| TEXAS INSTRUMENTS INCORPORATED
| Standard Linear and Logic Group
| IBIS Model of SN74CBTLV16211
| LOW-VOLTAGE 24-BIT FET BUS SWITCH
| This file contains package information for the following:
|  TVSOP 56-pin (DGV) package as [Component] CBTLV16211_DGV
|  TSSOP 56-pin (DGG) package as [Component] CBTLV16211_DGG
|  SSOP 56-pin (DL) package as [Component] CBTLV16211_DL
| This device can be powered at the following Vccs:
|  3.3 volt Vcc
|  2.5 volt Vcc
| This file provides unique models under the [Model Selector] for each Vcc.
| For operation at a specific Vcc, select the appropriate model after each
| [Model Selector] keyword.
[IBIS Ver]   3.2
[Comment char]  |_char
[File Name]   sn74cbtlv16211.ibs
[File Rev]   1.1 | b_die
[Date]   December 16, 2002
[Source]   Data created from TI-SPICE simulations at TI-SLL.
[Notes]   The following is an IBIS list for the CBTLV16211.
   Please contact sllibis@ti.com with questions and
   comments concerning SLL IBIS models.
   -Power clamp data deleted as there is no power-clamp diode.
   -Non-monotonic data due to FET characteristics.
[Disclaimer] Property of Texas Instruments Incorporated.  Unauthorized
   reproduction and/or distribution is strictly prohibited.
   This product is protected under copyright law.
   Created  2002, (C) Copyright  2002, Texas Instruments
   Incorporated, All Rights Reserved
   UNLESS THERE IS A SIGNED, WRITTEN AGREEMENT TO THE
   CONTRARY, TEXAS INSTRUMENTS (TI) IS PROVIDING THE IBIS
   MODELS  AND WITHOUT ANY WARRANTY, EXPRESSED OR
   IMPLIED.  TI assumes no liability for:
   1) the accuracy of the IBIS models provided to your
   company;
   2) the proper functioning of these IBIS Models in your
   design or for any resulting applications; or
   3) infringement of patents, copyrights or intellectual
   property rights resulting from your use of these IBIS
   models.
   TI provides IBIS Models as a service to our customers.
   You and your company shall not distribute, sell or give
   these models to anyone else without prior written
   permission from TI.
   TI reserves the right to make changes to our products or
   to discontinue any semiconductor product or service
   without notice, and advises our customers to obtain the
   latest version of relevant information to verify, before
   placing orders, that the information being relied on is
   current.
   Please be aware that your receipt and use of the IBIS
   information provided shall serve as acceptance of these
   terms and conditions.  If you do not accept these terms,
   you should return or destroy the IBIS models and any
   other accompanying information immediately.
| Component CBTLV16211_DGV 56-pin TVSOP
[Component]   CBTLV16211_DGV
[Manufacturer]   Texas Instruments, Inc.
[Package]
|   typ   min   max
R_pkg   6.300e-02   5.000e-02   8.600e-02
L_pkg   2.945e-09   2.392e-09   3.938e-09
C_pkg   3.910e-13   2.710e-13   5.880e-13
[Pin]   signal_name   model_name   R_pin   L_pin   C_pin
1   NC   NC   6.800e-02   3.933e-09   5.880e-13
2   1A1   CBTLV16211_IO   6.800e-02   3.569e-09   5.860e-13
3   1A2   CBTLV16211_IO   7.600e-02   3.464e-09   5.150e-13
4   1A3   CBTLV16211_IO   8.600e-02   3.451e-09   4.580e-13
5   1A4   CBTLV16211_IO   8.200e-02   3.278e-09   4.260e-13
6   1A5   CBTLV16211_IO   7.700e-02   3.143e-09   3.870e-13
7   1A6   CBTLV16211_IO   6.900e-02   2.971e-09   4.010e-13
8   GND   GND   5.000e-02   2.787e-09   3.790e-13
9   1A7   CBTLV16211_IO   5.100e-02   2.686e-09   3.200e-13
10   1A8   CBTLV16211_IO   5.200e-02   2.607e-09   3.160e-13
11   1A9   CBTLV16211_IO   5.300e-02   2.497e-09   2.970e-13
12   1A10   CBTLV16211_IO   5.400e-02   2.438e-09   2.920e-13
13   1A11   CBTLV16211_IO   5.500e-02   2.412e-09   2.860e-13
14   1A12   CBTLV16211_IO   5.500e-02   2.400e-09   2.730e-13
15   2A1   CBTLV16211_IO   5.500e-02   2.402e-09   2.730e-13
16   2A2   CBTLV16211_IO   5.400e-02   2.398e-09   2.840e-13
17   VCC   POWER   5.400e-02   2.407e-09   2.890e-13
18   2A3   CBTLV16211_IO   5.300e-02   2.448e-09   2.930e-13
19   GND   GND   5.200e-02   2.548e-09   3.110e-13
20   2A4   CBTLV16211_IO   5.100e-02   2.623e-09   3.160e-13
21   2A5   CBTLV16211_IO   5.000e-02   2.725e-09   3.700e-13
22   2A6   CBTLV16211_IO   6.500e-02   2.903e-09   3.940e-13
23   2A7   CBTLV16211_IO   7.300e-02   3.086e-09   3.870e-13
24   2A8   CBTLV16211_IO   8.200e-02   3.272e-09   4.280e-13
25   2A9   CBTLV16211_IO   8.200e-02   3.394e-09   4.570e-13
26   2A10   CBTLV16211_IO   7.100e-02   3.374e-09   5.080e-13
27   2A11   CBTLV16211_IO   6.900e-02   3.572e-09   5.810e-13
28   2A12   CBTLV16211_IO   6.900e-02   3.937e-09   5.740e-13
29   2B12   CBTLV16211_IO   6.900e-02   3.923e-09   5.690e-13
30   2B11   CBTLV16211_IO   6.800e-02   3.546e-09   5.740e-13
31   2B10   CBTLV16211_IO   7.400e-02   3.422e-09   5.180e-13
32   2B9   CBTLV16211_IO   8.100e-02   3.395e-09   4.680e-13
33   2B8   CBTLV16211_IO   8.000e-02   3.255e-09   4.310e-13
34   2B7   CBTLV16211_IO   7.100e-02   3.063e-09   3.860e-13
35   2B6   CBTLV16211_IO   6.100e-02   2.878e-09   3.900e-13
36   2B5   CBTLV16211_IO   5.000e-02   2.709e-09   3.640e-13
37   2B4   CBTLV16211_IO   5.100e-02   2.607e-09   3.110e-13
38   GND   GND   5.100e-02   2.532e-09   3.060e-13
39   2B3   CBTLV16211_IO   5.300e-02   2.440e-09   2.890e-13
40   2B2   CBTLV16211_IO   5.300e-02   2.399e-09   2.860e-13
41   2B1   CBTLV16211_IO   5.400e-02   2.392e-09   2.820e-13
42   1B12   CBTLV16211_IO   5.500e-02   2.399e-09   2.710e-13
43   1B11   CBTLV16211_IO   5.500e-02   2.395e-09   2.710e-13
44   1B10   CBTLV16211_IO   5.500e-02   2.403e-09   2.830e-13
45   1B9   CBTLV16211_IO   5.400e-02   2.421e-09   2.880e-13
46   1B8   CBTLV16211_IO   5.300e-02   2.472e-09   2.920e-13
47   1B7   CBTLV16211_IO   5.100e-02   2.569e-09   3.090e-13
48   1B6   CBTLV16211_IO   5.100e-02   2.636e-09   3.130e-13
49   GND   GND   5.000e-02   2.739e-09   3.660e-13
50   1B5   CBTLV16211_IO   6.500e-02   2.922e-09   3.900e-13
51   1B4   CBTLV16211_IO   7.200e-02   3.076e-09   3.840e-13
52   1B3   CBTLV16211_IO   8.100e-02   3.249e-09   4.300e-13
53   1B2   CBTLV16211_IO   8.300e-02   3.400e-09   4.550e-13
54   1B1   CBTLV16211_IO   7.300e-02   3.421e-09   5.060e-13
55   2NOE   CBTLV16211_NOE   6.900e-02   3.579e-09   5.780e-13
56   1NOE   CBTLV16211_NOE   6.900e-02   3.938e-09   5.810e-13
| Component CBTLV16211_DGG 56-pin TSSOP
[Component]   CBTLV16211_DGG
[Manufacturer]   Texas Instruments, Inc.
[Package]
|   typ   min   max
R_pkg   4.500e-02   3.500e-02   6.200e-02
L_pkg   3.324e-09   2.403e-09   5.094e-09
C_pkg   5.640e-13   3.410e-13   9.140e-13
[Pin]   signal_name   model_name   R_pin   L_pin   C_pin
1   NC   NC   6.200e-02   5.094e-09   8.560e-13
2   1A1   CBTLV16211_IO   6.100e-02   4.621e-09   9.020e-13
3   1A2   CBTLV16211_IO   6.000e-02   4.316e-09   8.020e-13
4   1A3   CBTLV16211_IO   5.900e-02   3.968e-09   6.980e-13
5   1A4   CBTLV16211_IO   5.700e-02   3.716e-09   6.490e-13
6   1A5   CBTLV16211_IO   4.200e-02   3.517e-09   6.520e-13
7   1A6   CBTLV16211_IO   4.100e-02   3.160e-09   5.700e-13
8   GND   GND   3.900e-02   2.981e-09   4.820e-13
9   1A7   CBTLV16211_IO   3.900e-02   2.809e-09   4.470e-13
10   1A8   CBTLV16211_IO   3.800e-02   2.715e-09   4.090e-13
11   1A9   CBTLV16211_IO   4.100e-02   2.675e-09   3.910e-13
12   1A10   CBTLV16211_IO   3.900e-02   2.536e-09   3.660e-13
13   1A11   CBTLV16211_IO   3.900e-02   2.457e-09   3.480e-13
14   1A12   CBTLV16211_IO   3.800e-02   2.411e-09   3.530e-13
15   2A1   CBTLV16211_IO   3.900e-02   2.456e-09   3.550e-13
16   2A2   CBTLV16211_IO   3.900e-02   2.471e-09   3.490e-13
17   VCC   POWER   4.000e-02   2.580e-09   3.700e-13
18   2A3   CBTLV16211_IO   3.800e-02   2.651e-09   3.890e-13
19   GND   GND   3.800e-02   2.739e-09   4.110e-13
20   2A4   CBTLV16211_IO   3.900e-02   2.838e-09   4.490e-13
21   2A5   CBTLV16211_IO   3.800e-02   2.988e-09   4.840e-13
22   2A6   CBTLV16211_IO   3.800e-02   3.105e-09   5.640e-13
23   2A7   CBTLV16211_IO   4.000e-02   3.427e-09   6.380e-13
24   2A8   CBTLV16211_IO   5.600e-02   3.654e-09   6.410e-13
25   2A9   CBTLV16211_IO   5.700e-02   3.932e-09   7.000e-13
26   2A10   CBTLV16211_IO   5.800e-02   4.257e-09   8.060e-13
27   2A11   CBTLV16211_IO   5.700e-02   4.580e-09   9.140e-13
28   2A12   CBTLV16211_IO   5.900e-02   5.038e-09   8.610e-13
29   2B12   CBTLV16211_IO   6.000e-02   5.058e-09   8.580e-13
30   2B11   CBTLV16211_IO   5.600e-02   4.543e-09   9.040e-13
31   2B10   CBTLV16211_IO   5.700e-02   4.240e-09   8.030e-13
32   2B9   CBTLV16211_IO   5.700e-02   3.929e-09   7.000e-13
33   2B8   CBTLV16211_IO   5.600e-02   3.616e-09   6.370e-13
34   2B7   CBTLV16211_IO   3.700e-02   3.368e-09   6.400e-13
35   2B6   CBTLV16211_IO   3.600e-02   3.024e-09   5.630e-13
36   2B5   CBTLV16211_IO   3.500e-02   2.876e-09   4.740e-13
37   2B4   CBTLV16211_IO   3.500e-02   2.745e-09   4.440e-13
38   GND   GND   3.700e-02   2.683e-09   4.050e-13
39   2B3   CBTLV16211_IO   3.800e-02   2.603e-09   3.820e-13
40   2B2   CBTLV16211_IO   3.800e-02   2.510e-09   3.620e-13
41   2B1   CBTLV16211_IO   3.600e-02   2.412e-09   3.410e-13
42   1B12   CBTLV16211_IO   3.800e-02   2.416e-09   3.490e-13
43   1B11   CBTLV16211_IO   3.700e-02   2.403e-09   3.490e-13
44   1B10   CBTLV16211_IO   3.700e-02   2.429e-09   3.410e-13
45   1B9   CBTLV16211_IO   3.600e-02   2.482e-09   3.580e-13
46   1B8   CBTLV16211_IO   3.700e-02   2.615e-09   3.810e-13
47   1B7   CBTLV16211_IO   3.500e-02   2.669e-09   4.020e-13
48   1B6   CBTLV16211_IO   3.600e-02   2.763e-09   4.420e-13
49   GND   GND   3.600e-02   2.942e-09   4.780e-13
50   1B5   CBTLV16211_IO   3.500e-02   3.053e-09   5.640e-13
51   1B4   CBTLV16211_IO   3.600e-02   3.409e-09   6.410e-13
52   1B3   CBTLV16211_IO   5.800e-02   3.698e-09   6.410e-13
53   1B2   CBTLV16211_IO   5.900e-02   3.975e-09   6.970e-13
54   1B1   CBTLV16211_IO   6.100e-02   4.327e-09   8.020e-13
55   2NOE   CBTLV16211_NOE   6.100e-02   4.624e-09   9.050e-13
56   1NOE   CBTLV16211_NOE   6.000e-02   5.063e-09   8.580e-13
| Component CBTLV16211_DL 56-pin SSOP
[Component]   CBTLV16211_DL
[Manufacturer]   Texas Instruments, Inc.
[Package]
|   typ   min   max
R_pkg   5.500e-02   4.800e-02   6.700e-02
L_pkg   6.539e-09   4.802e-09   9.746e-09
C_pkg   1.880e-13   7.600e-14   5.170e-13
[Pin]   signal_name   model_name   R_pin   L_pin   C_pin
1   NC   NC   6.400e-02   9.646e-09   5.130e-13
2   1A1   CBTLV16211_IO   5.900e-02   8.723e-09   2.700e-13
3   1A2   CBTLV16211_IO   5.900e-02   8.139e-09   2.230e-13
4   1A3   CBTLV16211_IO   5.600e-02   7.554e-09   2.010e-13
5   1A4   CBTLV16211_IO   5.400e-02   6.991e-09   1.950e-13
6   1A5   CBTLV16211_IO   5.300e-02   6.659e-09   2.020e-13
7   1A6   CBTLV16211_IO   5.500e-02   6.321e-09   2.070e-13
8   GND   GND   5.500e-02   5.942e-09   1.330e-13
9   1A7   CBTLV16211_IO   5.700e-02   5.767e-09   1.320e-13
10   1A8   CBTLV16211_IO   5.400e-02   5.459e-09   1.210e-13
11   1A9   CBTLV16211_IO   5.100e-02   5.224e-09   1.400e-13
12   1A10   CBTLV16211_IO   4.800e-02   5.088e-09   1.260e-13
13   1A11   CBTLV16211_IO   5.000e-02   5.021e-09   9.600e-14
14   1A12   CBTLV16211_IO   5.100e-02   4.802e-09   7.600e-14
15   2A1   CBTLV16211_IO   5.100e-02   4.803e-09   7.600e-14
16   2A2   CBTLV16211_IO   5.000e-02   5.021e-09   9.600e-14
17   VCC   POWER   4.800e-02   5.088e-09   1.260e-13
18   2A3   CBTLV16211_IO   5.100e-02   5.224e-09   1.400e-13
19   GND   GND   5.400e-02   5.459e-09   1.210e-13
20   2A4   CBTLV16211_IO   5.700e-02   5.768e-09   1.330e-13
21   2A5   CBTLV16211_IO   5.500e-02   5.942e-09   1.330e-13
22   2A6   CBTLV16211_IO   5.500e-02   6.320e-09   2.060e-13
23   2A7   CBTLV16211_IO   5.300e-02   6.659e-09   2.030e-13
24   2A8   CBTLV16211_IO   5.400e-02   6.991e-09   1.960e-13
25   2A9   CBTLV16211_IO   5.600e-02   7.554e-09   2.010e-13
26   2A10   CBTLV16211_IO   5.900e-02   8.139e-09   2.230e-13
27   2A11   CBTLV16211_IO   5.900e-02   8.727e-09   2.700e-13
28   2A12   CBTLV16211_IO   6.700e-02   9.746e-09   5.170e-13
29   2B12   CBTLV16211_IO   6.300e-02   9.630e-09   5.110e-13
30   2B11   CBTLV16211_IO   6.000e-02   8.751e-09   2.710e-13
31   2B10   CBTLV16211_IO   6.000e-02   8.184e-09   2.250e-13
32   2B9   CBTLV16211_IO   5.600e-02   7.543e-09   2.000e-13
33   2B8   CBTLV16211_IO   5.400e-02   7.005e-09   1.960e-13
34   2B7   CBTLV16211_IO   5.600e-02   6.714e-09   2.040e-13
35   2B6   CBTLV16211_IO   5.800e-02   6.384e-09   2.080e-13
36   2B5   CBTLV16211_IO   5.700e-02   5.976e-09   1.340e-13
37   2B4   CBTLV16211_IO   5.700e-02   5.743e-09   1.300e-13
38   GND   GND   5.400e-02   5.468e-09   1.190e-13
39   2B3   CBTLV16211_IO   5.500e-02   5.328e-09   1.420e-13
40   2B2   CBTLV16211_IO   5.200e-02   5.189e-09   1.290e-13
41   2B1   CBTLV16211_IO   5.200e-02   5.053e-09   9.600e-14
42   1B12   CBTLV16211_IO   5.100e-02   4.825e-09   7.600e-14
43   1B11   CBTLV16211_IO   5.400e-02   4.896e-09   7.800e-14
44   1B10   CBTLV16211_IO   5.200e-02   5.093e-09   9.700e-14
45   1B9   CBTLV16211_IO   5.100e-02   5.179e-09   1.280e-13
46   1B8   CBTLV16211_IO   5.400e-02   5.314e-09   1.420e-13
47   1B7   CBTLV16211_IO   5.500e-02   5.511e-09   1.210e-13
48   1B6   CBTLV16211_IO   5.700e-02   5.771e-09   1.310e-13
49   GND   GND   5.600e-02   5.957e-09   1.330e-13
50   1B5   CBTLV16211_IO   5.500e-02   6.320e-09   2.060e-13
51   1B4   CBTLV16211_IO   5.200e-02   6.621e-09   2.000e-13
52   1B3   CBTLV16211_IO   5.300e-02   6.973e-09   1.950e-13
53   1B2   CBTLV16211_IO   5.700e-02   7.571e-09   2.020e-13
54   1B1   CBTLV16211_IO   5.700e-02   8.097e-09   2.220e-13
55   2NOE   CBTLV16211_NOE   5.900e-02   8.723e-09   2.710e-13
56   1NOE   CBTLV16211_NOE   6.100e-02   9.560e-09   5.090e-13
[Series Switch Groups]
| Function Group States
On  1 /   | 1A1-1A12->1B1-1B12 1NOE LOW
On  2 /   | 2A1-2A12->2B1-2B12 2NOE LOW
On  1 2 /   | 1NOE, LOW, 2NOE, LOW
[Series Pin Mapping]   pin_2   model_name   function_table_group
2   54   CBTLV16211_IO_33_S   1
| 2   54   CBTLV16211_IO_25_S   1
3   53   CBTLV16211_IO_33_S   1
| 3   53   CBTLV16211_IO_25_S   1
4   52   CBTLV16211_IO_33_S   1
| 4   52   CBTLV16211_IO_25_S   1
5   51   CBTLV16211_IO_33_S   1
| 5   51   CBTLV16211_IO_25_S   1
6   50   CBTLV16211_IO_33_S   1
| 6   50   CBTLV16211_IO_25_S   1
7   48   CBTLV16211_IO_33_S   1
| 7   48   CBTLV16211_IO_25_S   1
9   47   CBTLV16211_IO_33_S   1
| 9   47   CBTLV16211_IO_25_S   1
10   46   CBTLV16211_IO_33_S   1
| 10   46   CBTLV16211_IO_25_S   1
11   45   CBTLV16211_IO_33_S   1
| 11   45   CBTLV16211_IO_25_S   1
12   44   CBTLV16211_IO_33_S   1
| 12   44   CBTLV16211_IO_25_S   1
13   43   CBTLV16211_IO_33_S   1
| 13   43   CBTLV16211_IO_25_S   1
14   42   CBTLV16211_IO_33_S   1
| 14   42   CBTLV16211_IO_25_S   1
15   41   CBTLV16211_IO_33_S   2
| 15   41   CBTLV16211_IO_25_S   2
16   40   CBTLV16211_IO_33_S   2
| 16   40   CBTLV16211_IO_25_S   2
18   39   CBTLV16211_IO_33_S   2
| 18   39   CBTLV16211_IO_25_S   2
20   37   CBTLV16211_IO_33_S   2
| 20   37   CBTLV16211_IO_25_S   2
21   36   CBTLV16211_IO_33_S   2
| 21   36   CBTLV16211_IO_25_S   2
22   35   CBTLV16211_IO_33_S   2
| 22   35   CBTLV16211_IO_25_S   2
23   34   CBTLV16211_IO_33_S   2
| 23   34   CBTLV16211_IO_25_S   2
24   33   CBTLV16211_IO_33_S   2
| 24   33   CBTLV16211_IO_25_S   2
25   32   CBTLV16211_IO_33_S   2
| 25   32   CBTLV16211_IO_25_S   2
26   31   CBTLV16211_IO_33_S   2
| 26   31   CBTLV16211_IO_25_S   2
27   30   CBTLV16211_IO_33_S   2
| 27   30   CBTLV16211_IO_25_S   2
28   29   CBTLV16211_IO_33_S   2
| 28   29   CBTLV16211_IO_25_S   2
| Model CBTLV16211_NOE
[Model Selector]   CBTLV16211_NOE
CBTLV16211_NOE_33   3.3 volt Vcc
CBTLV16211_NOE_25   2.5 volt Vcc
| Model CBTLV16211_IO
[Model Selector]   CBTLV16211_IO
CBTLV16211_IO_33   3.3 volt Vcc
CBTLV16211_IO_25   2.5 volt Vcc
| Model CBTLV16211_IO_S
[Model Selector]   CBTLV16211_IO_S
CBTLV16211_IO_33_S   3.3 volt Vcc
CBTLV16211_IO_25_S   2.5 volt Vcc
[Model]   CBTLV16211_IO_33_S
Model_type  Series_switch
| variable   typ   min   max
C_comp   0   0   0
[Temperature Range]   40   100   -40
| Ambient temperature   25   85   -40
[Voltage range]   3.3   3   3.6
[On]
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[Off]
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[Model]   CBTLV16211_IO_25_S
Model_type  Series_switch
| variable   typ   min   max
C_comp   0   0   0
[Temperature Range]   40   100   -40
| Ambient temperature   25   85   -40
[Voltage range]   2.5   2.3   2.7
[On]
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[Off]
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| Models and submodels in the file (6): CBTLV16211_NOE_33 (Input), CBTLV16211_NOE_25 (Input), CBTLV16211_IO_33_S (Series_switch), CBTLV16211_IO_33 (Terminator), CBTLV16211_IO_25_S (Series_switch), CBTLV16211_IO_25 (Terminator)
